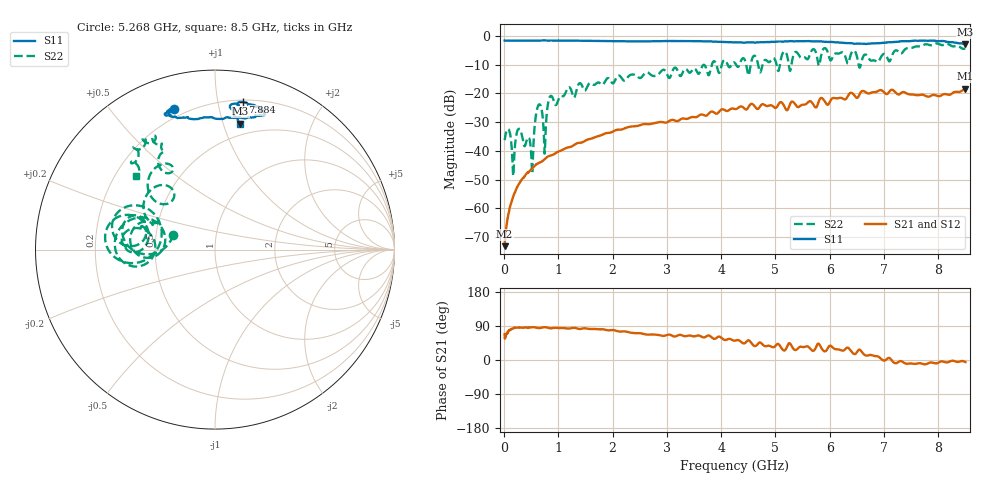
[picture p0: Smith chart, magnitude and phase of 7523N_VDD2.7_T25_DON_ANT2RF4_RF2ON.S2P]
!Agilent Technologies,E5071C,MY46417908,A.11.23
!Date: Wed Dec 09 17:50:09 2020
!Data & Calibration Information:
!Freq	S11:SOLT2(ON)	S21:SOLT2(ON)	S12:SOLT2(ON)	S22:SOLT2(ON)
!PortZ  Port1:50+j0  Port2:50+j0
!Above PortZ is port z conversion or system Z0 setting when saving the data.
!When reading, reference impedance value at option line is always used.
# Hz S dB R 50
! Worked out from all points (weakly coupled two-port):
!   1601 points, 10 MHz to 8.5 GHz, reference 50 ohm
!   highest |S21| = -18.34 dB at 8.5 GHz (marker M1); lowest = -73.2 dB at 10 MHz (marker M2)
!   lowest |S11| = -2.9 dB at 8.5 GHz (marker M3), VSWR 6.05, Z = 19.8 + j57.1 ohm
!   |S11| at or under -10 dB: nowhere
!   |S22| runs from -48.7 to -2.6 dB; largest |S21 - S12| = 0.001
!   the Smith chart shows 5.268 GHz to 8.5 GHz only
!   S11 on the Smith chart (normalised r, x): 5.268 GHz: 0.16, +0.74; 7.884 GHz: 0.22, +1.18; 8.5 GHz: 0.40, +1.14
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1e7  -1.56 179.7  -73.18 68.2  -72.58 63.5  -36.24 5.6
8.42875e7  -1.58 178.3  -61.70 77.4  -61.68 76.6  -32.50 -37.6
1.691875e8  -1.59 176.7  -55.90 83.4  -56.09 83.5  -48.73 165.7
2.647e8  -1.58 175.1  -51.78 85.4  -51.83 85.6  -32.40 -10.3
3.602125e8  -1.56 173.6  -49.41 85.5  -49.32 85.4  -37.64 -77.3
5.140938e8  -1.57 171.1  -46.17 86.4  -46.19 86.1  -46.64 -89.4
6.414438e8  -1.54 169.6  -44.18 84.2  -44.17 84.2  -23.85 -93.2
7.475688e8  -1.56 168.4  -42.85 86.6  -42.88 86.5  -40.97 -108.2
8.536938e8  -1.55 167.2  -41.62 83.6  -41.60 83.5  -20.91 -101.1
1.426769e9  -1.63 162.9  -37.10 82.6  -37.10 82.5  -16.91 -125.6
2.843538e9  -1.79 138.2  -30.01 65.9  -30.02 65.9  -13.32 -143.2
4.255e9  -2.17 126.2  -25.43 51.0  -25.42 51.0  -9.40 -151.8
5.050938e9  -1.89 106.7  -23.94 42.5  -23.94 42.5  -12.16 170.4
5.167675e9  -1.90 106.2  -24.65 25.1  -24.65 25.3  -5.33 164.2
5.268494e9  -1.76 106.1  -23.71 43.5  -23.73 43.6  -12.13 160.3
5.671769e9  -1.84 108.7  -23.13 25.4  -23.11 25.7  -4.95 172.4
5.793812e9  -1.83 108.6  -23.02 43.3  -23.06 43.4  -10.06 161.0
5.905244e9  -2.00 109.9  -22.66 22.9  -22.66 23.3  -4.20 173.3
6.382806e9  -2.46 101.6  -19.80 25.4  -19.85 25.4  -6.75 -168.2
7.088538e9  -2.16 73.3  -19.60 5.6  -19.64 5.6  -8.71 128.9
7.884475e9  -1.54 79.2  -20.63 -6.7  -20.63 -6.6  -3.15 121.6
8.5e9  -2.90 78.6  -18.34 -5.4  -18.34 -5.1  -4.43 136.9
